| IBIS file stm32h503_wlcsp25.ibs
[IBIS ver] 4.2
[File name] stm32h503_wlcsp25.ibs
[File Rev] 1.2
[Date] 07-05-2024
[Source] Data Created at STMicroelectronics
[Notes]  File originated from ELDO simulations.
[Disclaimer]  This information is for modeling purpose only and is
   not guaranteed. The information is subject to change without
   notice.
[Copyright] Copyright 2024 STMicroelectronics Inc.
|   Component stm32h503_wlcsp25
[Component] stm32h503_wlcsp25
[Manufacturer] STMicroelectronics
[Package]
| variable   typ   min   max
R_pkg  0  NA  NA
L_pkg  0  NA  NA
C_pkg  0  NA  NA
[Pin]   signal_name   model_name
A1  PA12  io8usb_ft_i3c_spi_phy
A2  PA15  io8_ft_i3c_spi
A3  BOOT0  io8_ft_i3c_spi
A4  PB7  io8_ft_i3c_spi
A5  PB8  io8_ft_i3c_spi
B1  PA11  io8usb_ft_i3c_spi_phy
B2  VDDIO2  power
B3  PB5  io8_ft_i3c_spi
B4  PB6  io8_ft_i3c_spi
B5  PC14-OSC32_IN  io_ft_tamp
C1  PA8  io8_ft_i3c_spi
C2  PA14  io8_ft_i3c_spi
C3  VSS  gnd
C4  PB4  io8_ft_i3c_spi
C5  PC15-OSC32_OUT  io_ft_tamp
D1  PA9  io8_ft_i3c_spi
D2  PA13  io8_ft_i3c_spi
D3  PB3  io8_ft_i3c_spi
D4  VDD  power
D5  NRST  ioreset_ft_v33
E1  PB15  io8_ft_spi
E2  VCAP  nc
E3  PA7  io8_ft_spi
E4  PA5  io8_ft_spi
E5  PA0  io8_ft_spi
[Package Model]   474-wlcsp-25-100mhz-221024
[Pin Mapping]   pulldown_ref   pullup_ref   | Comment
A1  gndio  vddio
A2  gndio  vddio  | Depending on IO usage
| A2  gndio  vddio2  | Depending on IO usage
A3  gndio  vddio
A4  gndio  vddio  | Depending on IO usage
| A4  gndio  vddio2  | Depending on IO usage
A5  gndio  vddio  | Depending on IO usage
| A5  gndio  vddio2  | Depending on IO usage
B1  gndio  vddio
B2  nc  vddio2
B3  gndio  vddio  | Depending on IO usage
| B3  gndio  vddio2  | Depending on IO usage
B4  gndio  vddio  | Depending on IO usage
| B4  gndio  vddio2  | Depending on IO usage
B5  gndio  vddio
C1  gndio  vddio  | Depending on IO usage
| C1  gndio  vddio2  | Depending on IO usage
C2  gndio  vddio
C3  gndio  nc
C4  gndio  vddio  | Depending on IO usage
| C4  gndio  vddio2  | Depending on IO usage
C5  gndio  vddio
D1  gndio  vddio  | Depending on IO usage
| D1  gndio  vddio2  | Depending on IO usage
D2  gndio  vddio
D3  gndio  vddio  | Depending on IO usage
| D3  gndio  vddio2  | Depending on IO usage
D4  nc  vddio
D5  gndio  vddio
E1  gndio  vddio  | Depending on IO usage
| E1  gndio  vddio2  | Depending on IO usage
E2  nc  nc
E3  gndio  vddio
E4  gndio  vddio
E5  gndio  vddio
[Model Selector] io8_ft_i3c_spi
io8_ft_spi_ls_1v2 "GPIO SPI - 5V tolerant - low speed - 1.2V range"
io8_ft_spi_ls_1v8 "GPIO SPI - 5V tolerant - low speed - 1.8V range"
io8_ft_spi_ls_3v3 "GPIO SPI - 5V tolerant - low speed - 3.3V range"
io8_ft_spi_ms_1v2 "GPIO SPI - 5V tolerant - med speed - 1.2V range"
io8_ft_spi_ms_1v8 "GPIO SPI - 5V tolerant - med speed - 1.8V range"
io8_ft_spi_ms_3v3 "GPIO SPI - 5V tolerant - med speed - 3.3V range"
io8_ft_spi_fs_1v2 "GPIO SPI - 5V tolerant - fast speed - 1.2V range"
io8_ft_spi_fs_1v8 "GPIO SPI - 5V tolerant - fast speed - 1.8V range"
io8_ft_spi_fs_3v3 "GPIO SPI - 5V tolerant - fast speed - 3.3V range"
io8_ft_spi_hs_1v2 "GPIO SPI - 5V tolerant - high speed - 1.2V range"
io8_ft_spi_hs_1v8 "GPIO SPI - 5V tolerant - high speed - 1.8V range"
io8_ft_spi_hs_3v3 "GPIO SPI - 5V tolerant - high speed - 3.3V range"
io8_ft_hslv_spi_ls_1v2 "GPIO SPI low volt opt - 5V tolerant - low speed - 1.2V range"
io8_ft_hslv_spi_ls_1v8 "GPIO SPI low volt opt - 5V tolerant - low speed - 1.8V range"
io8_ft_hslv_spi_ls_2v5 "GPIO SPI low volt opt - 5V tolerant - low speed - 2.5V range"
io8_ft_hslv_spi_ms_1v2 "GPIO SPI low volt opt - 5V tolerant - med speed - 1.2V range"
io8_ft_hslv_spi_ms_1v8 "GPIO SPI low volt opt - 5V tolerant - med speed - 1.8V range"
io8_ft_hslv_spi_ms_2v5 "GPIO SPI low volt opt - 5V tolerant - med speed - 2.5V range"
io8_ft_hslv_spi_fs_1v2 "GPIO SPI low volt opt - 5V tolerant - fast speed - 1.2V range"
io8_ft_hslv_spi_fs_1v8 "GPIO SPI low volt opt - 5V tolerant - fast speed - 1.8V range"
io8_ft_hslv_spi_fs_2v5 "GPIO SPI low volt opt - 5V tolerant - fast speed - 2.5V range"
io8_ft_hslv_spi_hs_1v2 "GPIO SPI low volt opt - 5V tolerant - high speed - 1.2V range"
io8_ft_hslv_spi_hs_1v8 "GPIO SPI low volt opt - 5V tolerant - high speed - 1.8V range"
io8_ft_hslv_spi_hs_2v5 "GPIO SPI low volt opt - 5V tolerant - high speed - 2.5V range"
io8_ft_i3c_spi_ls_1v2 "GPIO SPI with I3C open-drain - 5V tolerant - low speed - 1.2V range"
io8_ft_i3c_spi_ls_1v8 "GPIO SPI with I3C open-drain - 5V tolerant - low speed - 1.8V range"
io8_ft_i3c_spi_ls_3v3 "GPIO SPI with I3C open-drain - 5V tolerant - low speed - 3.3V range"
io8_ft_i3c_spi_ms_1v2 "GPIO SPI with I3C open-drain - 5V tolerant - med speed - 1.2V range"
io8_ft_i3c_spi_ms_1v8 "GPIO SPI with I3C open-drain - 5V tolerant - med speed - 1.8V range"
io8_ft_i3c_spi_ms_3v3 "GPIO SPI with I3C open-drain - 5V tolerant - med speed - 3.3V range"
io8_ft_i3c_spi_fs_1v2 "GPIO SPI with I3C open-drain - 5V tolerant - fast speed - 1.2V range"
io8_ft_i3c_spi_fs_1v8 "GPIO SPI with I3C open-drain - 5V tolerant - fast speed - 1.8V range"
io8_ft_i3c_spi_fs_3v3 "GPIO SPI with I3C open-drain - 5V tolerant - fast speed - 3.3V range"
io8_ft_i3c_spi_hs_1v2 "GPIO SPI with I3C open-drain - 5V tolerant - high speed - 1.2V range"
io8_ft_i3c_spi_hs_1v8 "GPIO SPI with I3C open-drain - 5V tolerant - high speed - 1.8V range"
io8_ft_i3c_spi_hs_3v3 "GPIO SPI with I3C open-drain - 5V tolerant - high speed - 3.3V range"
io8_ft_hslv_i3c_spi_ls_1v2 "GPIO SPI low volt opt with I3C open-drain - 5V tolerant - low speed - 1.2V range"
io8_ft_hslv_i3c_spi_ls_1v8 "GPIO SPI low volt opt with I3C open-drain - 5V tolerant - low speed - 1.8V range"
io8_ft_hslv_i3c_spi_ls_2v5 "GPIO SPI low volt opt with I3C open-drain - 5V tolerant - low speed - 2.5V range"
io8_ft_hslv_i3c_spi_ms_1v2 "GPIO SPI low volt opt with I3C open-drain - 5V tolerant - med speed - 1.2V range"
io8_ft_hslv_i3c_spi_ms_1v8 "GPIO SPI low volt opt with I3C open-drain - 5V tolerant - med speed - 1.8V range"
io8_ft_hslv_i3c_spi_ms_2v5 "GPIO SPI low volt opt with I3C open-drain - 5V tolerant - med speed - 2.5V range"
io8_ft_hslv_i3c_spi_fs_1v2 "GPIO SPI low volt opt with I3C open-drain - 5V tolerant - fast speed - 1.2V range"
io8_ft_hslv_i3c_spi_fs_1v8 "GPIO SPI low volt opt with I3C open-drain - 5V tolerant - fast speed - 1.8V range"
io8_ft_hslv_i3c_spi_fs_2v5 "GPIO SPI low volt opt with I3C open-drain - 5V tolerant - fast speed - 2.5V range"
io8_ft_hslv_i3c_spi_hs_1v2 "GPIO SPI low volt opt with I3C open-drain - 5V tolerant - high speed - 1.2V range"
io8_ft_hslv_i3c_spi_hs_1v8 "GPIO SPI low volt opt with I3C open-drain - 5V tolerant - high speed - 1.8V range"
io8_ft_hslv_i3c_spi_hs_2v5 "GPIO SPI low volt opt with I3C open-drain - 5V tolerant - high speed - 2.5V range"
io8_ft_i3c_fmp_spi_3v3 "GPIO SPI with I3C fm+ open-drain - 5V tolerant - 3.3V range"
io8_ft_i3c_fmp_spi_1v8 "GPIO SPI with I3C fm+ open-drain - 5V tolerant - 1.8V range"
io8_ft_i3c_fmp_spi_1v2 "GPIO SPI with I3C fm+ open-drain - 5V tolerant - 1.2V range"
[Model Selector] io8_ft_spi
io8_ft_spi_ls_1v2 "GPIO SPI - 5V tolerant - low speed - 1.2V range"
io8_ft_spi_ls_1v8 "GPIO SPI - 5V tolerant - low speed - 1.8V range"
io8_ft_spi_ls_3v3 "GPIO SPI - 5V tolerant - low speed - 3.3V range"
io8_ft_spi_ms_1v2 "GPIO SPI- 5V tolerant - med speed - 1.2V range"
io8_ft_spi_ms_1v8 "GPIO SPI- 5V tolerant - med speed - 1.8V range"
io8_ft_spi_ms_3v3 "GPIO SPI- 5V tolerant - med speed - 3.3V range"
io8_ft_spi_fs_1v2 "GPIO SPI- 5V tolerant - fast speed - 1.2V range"
io8_ft_spi_fs_1v8 "GPIO SPI- 5V tolerant - fast speed - 1.8V range"
io8_ft_spi_fs_3v3 "GPIO SPI- 5V tolerant - fast speed - 3.3V range"
io8_ft_spi_hs_1v2 "GPIO SPI- 5V tolerant - high speed - 1.2V range"
io8_ft_spi_hs_1v8 "GPIO SPI- 5V tolerant - high speed - 1.8V range"
io8_ft_spi_hs_3v3 "GPIO SPI- 5V tolerant - high speed - 3.3V range"
io8_ft_hslv_spi_ls_1v2 "GPIO SPI low volt opt - 5V tolerant - low speed - 1.2V range"
io8_ft_hslv_spi_ls_1v8 "GPIO SPI low volt opt - 5V tolerant - low speed - 1.8V range"
io8_ft_hslv_spi_ls_2v5 "GPIO SPI low volt opt - 5V tolerant - low speed - 2.5V range"
io8_ft_hslv_spi_ms_1v2 "GPIO SPI low volt opt - 5V tolerant - med speed - 1.2V range"
io8_ft_hslv_spi_ms_1v8 "GPIO SPI low volt opt - 5V tolerant - med speed - 1.8V range"
io8_ft_hslv_spi_ms_2v5 "GPIO SPI low volt opt - 5V tolerant - med speed - 2.5V range"
io8_ft_hslv_spi_fs_1v2 "GPIO SPI low volt opt - 5V tolerant - fast speed - 1.2V range"
io8_ft_hslv_spi_fs_1v8 "GPIO SPI low volt opt - 5V tolerant - fast speed - 1.8V range"
io8_ft_hslv_spi_fs_2v5 "GPIO SPI low volt opt - 5V tolerant - fast speed - 2.5V range"
io8_ft_hslv_spi_hs_1v2 "GPIO SPI low volt opt - 5V tolerant - high speed - 1.2V range"
io8_ft_hslv_spi_hs_1v8 "GPIO SPI low volt opt - 5V tolerant - high speed - 1.8V range"
io8_ft_hslv_spi_hs_2v5 "GPIO SPI low volt opt - 5V tolerant - high speed - 2.5V range"
[Model Selector] io8usb_ft_i3c_spi_phy
io8_ft_spi_ls_1v2 "GPIO SPI - 5V tolerant - low speed - 1.2V range"
io8_ft_spi_ls_1v8 "GPIO SPI - 5V tolerant - low speed - 1.8V range"
io8_ft_spi_ls_3v3 "GPIO SPI - 5V tolerant - low speed - 3.3V range"
io8_ft_spi_ms_1v2 "GPIO SPI - 5V tolerant - med speed - 1.2V range"
io8_ft_spi_ms_1v8 "GPIO SPI - 5V tolerant - med speed - 1.8V range"
io8_ft_spi_ms_3v3 "GPIO SPI - 5V tolerant - med speed - 3.3V range"
io8_ft_spi_fs_1v2 "GPIO SPI - 5V tolerant - fast speed - 1.2V range"
io8_ft_spi_fs_1v8 "GPIO SPI - 5V tolerant - fast speed - 1.8V range"
io8_ft_spi_fs_3v3 "GPIO SPI - 5V tolerant - fast speed - 3.3V range"
io8_ft_spi_hs_1v2 "GPIO SPI - 5V tolerant - high speed - 1.2V range"
io8_ft_spi_hs_1v8 "GPIO SPI - 5V tolerant - high speed - 1.8V range"
io8_ft_spi_hs_3v3 "GPIO SPI - 5V tolerant - high speed - 3.3V range"
io8_ft_hslv_spi_ls_1v2 "GPIO SPI low volt opt - 5V tolerant - low speed - 1.2V range"
io8_ft_hslv_spi_ls_1v8 "GPIO SPI low volt opt - 5V tolerant - low speed - 1.8V range"
io8_ft_hslv_spi_ls_2v5 "GPIO SPI low volt opt - 5V tolerant - low speed - 2.5V range"
io8_ft_hslv_spi_ms_1v2 "GPIO SPI low volt opt - 5V tolerant - med speed - 1.2V range"
io8_ft_hslv_spi_ms_1v8 "GPIO SPI low volt opt - 5V tolerant - med speed - 1.8V range"
io8_ft_hslv_spi_ms_2v5 "GPIO SPI low volt opt - 5V tolerant - med speed - 2.5V range"
io8_ft_hslv_spi_fs_1v2 "GPIO SPI low volt opt - 5V tolerant - fast speed - 1.2V range"
io8_ft_hslv_spi_fs_1v8 "GPIO SPI low volt opt - 5V tolerant - fast speed - 1.8V range"
io8_ft_hslv_spi_fs_2v5 "GPIO SPI low volt opt - 5V tolerant - fast speed - 2.5V range"
io8_ft_hslv_spi_hs_1v2 "GPIO SPI low volt opt - 5V tolerant - high speed - 1.2V range"
io8_ft_hslv_spi_hs_1v8 "GPIO SPI low volt opt - 5V tolerant - high speed - 1.8V range"
io8_ft_hslv_spi_hs_2v5 "GPIO SPI low volt opt - 5V tolerant - high speed - 2.5V range"
io8_ft_i3c_spi_ls_1v2 "GPIO SPI  with I3C open-drain - 5V tolerant - low speed - 1.2V range"
io8_ft_i3c_spi_ls_1v8 "GPIO SPI  with I3C open-drain - 5V tolerant - low speed - 1.8V range"
io8_ft_i3c_spi_ls_3v3 "GPIO SPI  with I3C open-drain - 5V tolerant - low speed - 3.3V range"
io8_ft_i3c_spi_ms_1v2 "GPIO SPI  with I3C open-drain - 5V tolerant - med speed - 1.2V range"
io8_ft_i3c_spi_ms_1v8 "GPIO SPI  with I3C open-drain - 5V tolerant - med speed - 1.8V range"
io8_ft_i3c_spi_ms_3v3 "GPIO SPI  with I3C open-drain - 5V tolerant - med speed - 3.3V range"
io8_ft_i3c_spi_fs_1v2 "GPIO SPI  with I3C open-drain - 5V tolerant - fast speed - 1.2V range"
io8_ft_i3c_spi_fs_1v8 "GPIO SPI  with I3C open-drain - 5V tolerant - fast speed - 1.8V range"
io8_ft_i3c_spi_fs_3v3 "GPIO SPI  with I3C open-drain - 5V tolerant - fast speed - 3.3V range"
io8_ft_i3c_spi_hs_1v2 "GPIO SPI  with I3C open-drain - 5V tolerant - high speed - 1.2V range"
io8_ft_i3c_spi_hs_1v8 "GPIO SPI  with I3C open-drain - 5V tolerant - high speed - 1.8V range"
io8_ft_i3c_spi_hs_3v3 "GPIO SPI  with I3C open-drain - 5V tolerant - high speed - 3.3V range"
io8_ft_hslv_i3c_spi_ls_1v2 "GPIO SPI  low volt opt with I3C open-drain - 5V tolerant - low speed - 1.2V range"
io8_ft_hslv_i3c_spi_ls_1v8 "GPIO SPI  low volt opt with I3C open-drain - 5V tolerant - low speed - 1.8V range"
io8_ft_hslv_i3c_spi_ls_2v5 "GPIO SPI  low volt opt with I3C open-drain - 5V tolerant - low speed - 2.5V range"
io8_ft_hslv_i3c_spi_ms_1v2 "GPIO SPI  low volt opt with I3C open-drain - 5V tolerant - med speed - 1.2V range"
io8_ft_hslv_i3c_spi_ms_1v8 "GPIO SPI  low volt opt with I3C open-drain - 5V tolerant - med speed - 1.8V range"
io8_ft_hslv_i3c_spi_ms_2v5 "GPIO SPI  low volt opt with I3C open-drain - 5V tolerant - med speed - 2.5V range"
io8_ft_hslv_i3c_spi_fs_1v2 "GPIO SPI  low volt opt with I3C open-drain - 5V tolerant - fast speed - 1.2V range"
io8_ft_hslv_i3c_spi_fs_1v8 "GPIO SPI  low volt opt with I3C open-drain - 5V tolerant - fast speed - 1.8V range"
io8_ft_hslv_i3c_spi_fs_2v5 "GPIO SPI  low volt opt with I3C open-drain - 5V tolerant - fast speed - 2.5V range"
io8_ft_hslv_i3c_spi_hs_1v2 "GPIO SPI  low volt opt with I3C open-drain - 5V tolerant - high speed - 1.2V range"
io8_ft_hslv_i3c_spi_hs_1v8 "GPIO SPI  low volt opt with I3C open-drain - 5V tolerant - high speed - 1.8V range"
io8_ft_hslv_i3c_spi_hs_2v5 "GPIO SPI  low volt opt with I3C open-drain - 5V tolerant - high speed - 2.5V range"
io8_ft_i3c_fmp_spi_3v3 "GPIO SPI  with I3C fm+ open-drain - 5V tolerant - 3.3V range"
io8_ft_i3c_fmp_spi_1v8 "GPIO SPI  with I3C fm+ open-drain - 5V tolerant - 1.8V range"
io8_ft_i3c_fmp_spi_1v2 "GPIO SPI  with I3C fm+ open-drain - 5V tolerant - 1.2V range"
io8usb_ft_phy_ls_2v5 "USB PHY - 5V tolerant - low speed - 2.5V range"
io8usb_ft_phy_ls_3v3 "USB PHY - 5V tolerant - low speed - 3.3V range
io8usb_ft_phy_fs_2v5 "USB PHY - 5V tolerant - fast speed - 2.5V range"
io8usb_ft_phy_fs_3v3 "USB PHY - 5V tolerant - fast speed - 3.3V range"
[Model Selector] io_ft_tamp
io_ft_tamp_3v3 "IO tamper - 5V tolerant - 3.3V range"
io_ft_tamp_1v8 "IO tamper - 5V tolerant - 1.8V range"
io_ft_tamp_1v2 "IO tamper - 5V tolerant - 1.2V range"
[Model Selector] ioreset_ft_v33
ioreset_ft_v33_1v2 "Reset PAD. 5V tolerant. 1.2V range"
ioreset_ft_v33_1v8 "Reset PAD. 5V tolerant. 1.8V range"
ioreset_ft_v33_3v3 "Reset PAD. 5V tolerant. 3.3V range"
[Define Package Model]  474-wlcsp-25-100mhz-221024
[Manufacturer]  Unknown
[OEM]  Unknown
[Description]  None
[Number Of Pins]  25
[Pin Numbers]
| Pin Num   Terminal Name
A3 | BOOT0
D5 | NRST
E5 | PA0
E4 | PA5
E3 | PA7
C1 | PA8
D1 | PA9
B1 | PA11
A1 | PA12
D2 | PA13
C2 | PA14
A2 | PA15
D3 | PB3
C4 | PB4
B3 | PB5
B4 | PB6
A4 | PB7
A5 | PB8
E1 | PB15
B5 | PC14-OSC32_IN
C5 | PC15-OSC32_OUT
E2 | VCAP
D4 | VDD
B2 | VDDIO2
C3 | VSS
[Model Data]
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[End Model Data]
[End Package Model]
|End [Component]
| Models and submodels in the file (61): io8_ft_hslv_i3c_spi_fs_1v2 (I/O_open_drain), io8_ft_hslv_i3c_spi_fs_1v8 (I/O_open_drain), io8_ft_hslv_i3c_spi_fs_2v5 (I/O_open_drain), io8_ft_hslv_i3c_spi_hs_1v2 (I/O_open_drain), io8_ft_hslv_i3c_spi_hs_1v8 (I/O_open_drain), io8_ft_hslv_i3c_spi_hs_2v5 (I/O_open_drain), io8_ft_hslv_i3c_spi_ls_1v2 (I/O_open_drain), io8_ft_hslv_i3c_spi_ls_1v8 (I/O_open_drain), io8_ft_hslv_i3c_spi_ls_2v5 (I/O_open_drain), io8_ft_hslv_i3c_spi_ms_1v2 (I/O_open_drain), io8_ft_hslv_i3c_spi_ms_1v8 (I/O_open_drain), io8_ft_hslv_i3c_spi_ms_2v5 (I/O_open_drain), io8_ft_hslv_spi_fs_1v2 (I/O), io8_ft_hslv_spi_fs_1v8 (I/O), io8_ft_hslv_spi_fs_2v5 (I/O), io8_ft_hslv_spi_hs_1v2 (I/O), io8_ft_hslv_spi_hs_1v8 (I/O), io8_ft_hslv_spi_hs_2v5 (I/O), io8_ft_hslv_spi_ls_1v2 (I/O), io8_ft_hslv_spi_ls_1v8 (I/O), io8_ft_hslv_spi_ls_2v5 (I/O), io8_ft_hslv_spi_ms_1v2 (I/O), io8_ft_hslv_spi_ms_1v8 (I/O), io8_ft_hslv_spi_ms_2v5 (I/O), io8_ft_i3c_fmp_spi_1v2 (I/O_open_drain), io8_ft_i3c_fmp_spi_1v8 (I/O_open_drain), io8_ft_i3c_fmp_spi_3v3 (I/O_open_drain), io8_ft_i3c_spi_fs_1v2 (I/O_open_drain), io8_ft_i3c_spi_fs_1v8 (I/O_open_drain), io8_ft_i3c_spi_fs_3v3 (I/O_open_drain), io8_ft_i3c_spi_hs_1v2 (I/O_open_drain), io8_ft_i3c_spi_hs_1v8 (I/O_open_drain), io8_ft_i3c_spi_hs_3v3 (I/O_open_drain), io8_ft_i3c_spi_ls_1v2 (I/O_open_drain), io8_ft_i3c_spi_ls_1v8 (I/O_open_drain), io8_ft_i3c_spi_ls_3v3 (I/O_open_drain), io8_ft_i3c_spi_ms_1v2 (I/O_open_drain), io8_ft_i3c_spi_ms_1v8 (I/O_open_drain), io8_ft_i3c_spi_ms_3v3 (I/O_open_drain), io8_ft_spi_fs_1v2 (I/O), io8_ft_spi_fs_1v8 (I/O), io8_ft_spi_fs_3v3 (I/O), io8_ft_spi_hs_1v2 (I/O), io8_ft_spi_hs_1v8 (I/O), io8_ft_spi_hs_3v3 (I/O), io8_ft_spi_ls_1v2 (I/O), io8_ft_spi_ls_1v8 (I/O), io8_ft_spi_ls_3v3 (I/O), io8_ft_spi_ms_1v2 (I/O), io8_ft_spi_ms_1v8 (I/O), io8_ft_spi_ms_3v3 (I/O), io8usb_ft_phy_fs_2v5 (I/O), io8usb_ft_phy_fs_3v3 (I/O), io8usb_ft_phy_ls_2v5 (I/O), io8usb_ft_phy_ls_3v3 (I/O), io_ft_tamp_1v2 (I/O), io_ft_tamp_1v8 (I/O), io_ft_tamp_3v3 (I/O), ioreset_ft_v33_1v2 (I/O_open_drain), ioreset_ft_v33_1v8 (I/O_open_drain), ioreset_ft_v33_3v3 (I/O_open_drain)
